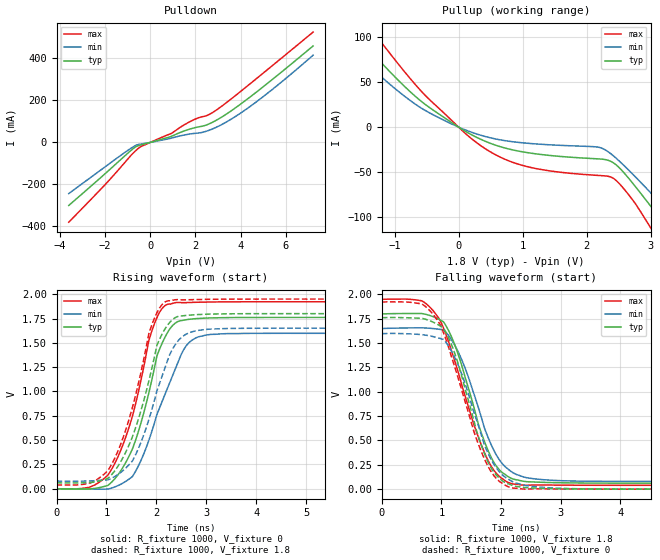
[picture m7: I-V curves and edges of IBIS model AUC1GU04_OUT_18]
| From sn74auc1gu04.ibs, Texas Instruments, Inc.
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[Model]   AUC1GU04_OUT_18
Model_type  Output
Vref =   0
Rref =   1000
Cref =   30p
Vmeas =   0.9
| variable   typ   min   max
C_comp   4.04pF   2.30pF   5.48pF
| C_pullup   3.63pF   2.30pF   4.77pF
| C_pulldown   4.44pF   3.81pF   5.48pF
[Temperature Range]   40   100   -40
| Ambient temperature   25   85   -40
[Voltage range]   1.8   1.65   1.95
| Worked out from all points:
|   slope of the pulldown table from 0 to 0.27 V, typ, clamps not added: 34.3 ohm
|   slope of the pullup table from 0 to 0.27 V, typ, clamps not added: 24.7 ohm
|   rising waveform, R_fixture 1000, V_fixture 0: 20-80 % time 574ps typ, 700ps min, 580ps max; typ from 0 V to 1.76 V
|   falling waveform, R_fixture 1000, V_fixture 1.8: 20-80 % time 532ps typ, 549ps min, 602ps max; typ from 1.8 V to 0.061 V
|   rising waveform, R_fixture 1000, V_fixture 1.8: 20-80 % time 585ps typ, 612ps min, 581ps max; typ from 0.061 V to 1.8 V
|   falling waveform, R_fixture 1000, V_fixture 0: 20-80 % time 515ps typ, 543ps min, 593ps max; typ from 1.76 V to 0 V
[Pulldown]
| AUC1GU04_OUT_18
|   Voltage   I(typ)   I(min)   I(max)
-3.6V     -299.9mA   -243.4mA   -379.6mA
-2.005V   -150mA     -117.1mA   -202.1mA
-1.075V   -59.54mA   -44.23mA   -89.65mA
-505mV    -14.41mA   -9.456mA   -26.45mA
930mV     28.79mA    20.33mA    42.75mA
1.695V    61.58mA    39.22mA    95.47mA
2.305V    77.38mA    48.04mA    122.5mA
2.625V    89.41mA    58.85mA    134.2mA
3.105V    117.1mA    81.96mA    168mA
3.865V    172.1mA    130.3mA    231.4mA
4.77V     246mA      199.5mA    310.3mA
7.2V      459.3mA    415.3mA    525.3mA
[Pullup]
| AUC1GU04_OUT_18
|   Voltage   I(typ)   I(min)   I(max)
-3.6V     272.1mA    245.4mA    305.2mA
-2.08V    141.8mA    117.9mA    173.1mA
-1.705V   110.8mA    89.81mA    139.4mA
-1.47V    91.91mA    73.25mA    118.1mA
-615mV    30.49mA    22.57mA    42.36mA
385mV     -14.76mA   -9.808mA   -22.53mA
1.135V    -28.98mA   -18.27mA   -44.95mA
2.365V    -37.66mA   -28.86mA   -55.16mA
2.945V    -82.69mA   -68.76mA   -105.6mA
3.13V     -99.83mA   -82.68mA   -126.8mA
3.49V     -133.6mA   -110.4mA   -168.3mA
7.2V      -482.6mA   -404.9mA   -584.6mA
[Ramp]
| AUC1GU04_OUT_18
| variable   typ   min   max
dV/dt_r   1.06/6.06E-10   0.96/7.50E-10   1.15/6.34E-10
dV/dt_f   1.05/5.81E-10   0.95/6.21E-10   1.15/6.22E-10
R_load = 1000
[Rising Waveform]
| AUC1GU04_OUT_18
R_fixture =   1000
C_fixture =   0
L_fixture =   0
V_fixture =   0
V_fixture_min = 0
V_fixture_max = 0
|   Time   V(typ)   V(min)   V(max)
0s        3.704nV    5.728nV    29.97nV
770ps     3.914mV    -4.412mV   40.57mV
1.24ns    150.5mV    34.44mV    340.5mV
1.58ns    496.4mV    177.7mV    868mV
1.955ns   1.231V     668.1mV    1.69V
2.14ns    1.526V     930.6mV    1.868V
2.4ns     1.711V     1.26V      1.915V
2.745ns   1.747V     1.538V     1.916V
3.425ns   1.759V     1.595V     1.921V
34.99ns   1.761V     1.597V     1.922V
[Falling Waveform]
| AUC1GU04_OUT_18
R_fixture =   1000
C_fixture =   0
L_fixture =   0
V_fixture =   1.8
V_fixture_min = 1.65
V_fixture_max = 1.95
|   Time   V(typ)   V(min)   V(max)
0s        1.8V       1.65V      1.95V
670ps     1.804V     1.657V     1.935V
1.035ns   1.718V     1.636V     1.654V
1.195ns   1.527V     1.508V     1.372V
1.355ns   1.241V     1.307V     1.042V
1.625ns   656.2mV    827.1mV    524.8mV
1.785ns   392.9mV    527.4mV    289.7mV
2.03ns    166mV      255.2mV    103.3mV
2.365ns   81.69mV    127.4mV    41.31mV
34.99ns   61.05mV    78.75mV    39.07mV
[Rising Waveform]
| AUC1GU04_OUT_18
R_fixture =   1000
C_fixture =   0
L_fixture =   0
V_fixture =   1.8
V_fixture_min = 1.65
V_fixture_max = 1.95
|   Time   V(typ)   V(min)   V(max)
0s        61.05mV    78.75mV    39.07mV
730ps     67.34mV    81.79mV    72mV
1.185ns   197.7mV    131.4mV    336mV
1.535ns   556.9mV    301.1mV    866.9mV
1.93ns    1.288V     853.9mV    1.716V
2.095ns   1.572V     1.132V     1.882V
2.39ns    1.763V     1.492V     1.944V
2.785ns   1.789V     1.623V     1.945V
3.81ns    1.8V       1.65V      1.95V
34.99ns   1.8V       1.65V      1.95V
[Falling Waveform]
| AUC1GU04_OUT_18
R_fixture =   1000
C_fixture =   0
L_fixture =   0
V_fixture =   0
V_fixture_min = 0
V_fixture_max = 0
|   Time   V(typ)   V(min)   V(max)
0s        1.761V     1.597V     1.922V
670ps     1.755V     1.587V     1.902V
880ps     1.71V      1.564V     1.779V
1.035ns   1.653V     1.538V     1.606V
1.315ns   1.217V     1.222V     1.07V
1.55ns    691.4mV    781.4mV    581.8mV
1.77ns    292.6mV    384.2mV    247.4mV
2.015ns   88.66mV    149.7mV    61.71mV
2.35ns    19.74mV    45.67mV    2.045mV
34.99ns   71.35nV    54.11nV    52.34nV
